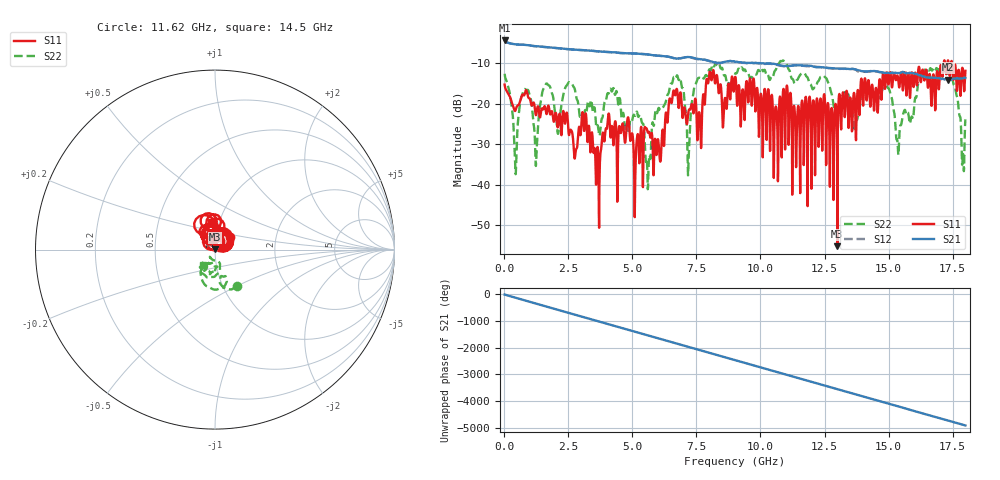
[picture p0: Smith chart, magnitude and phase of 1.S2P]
!Agilent Technologies,E5071C,MY46316741,A.11.02
!Date: Thu Sep 29 15:38:55 2022
!Data & Calibration Information:
!Freq	S11:SOLT2(ON)	S21:SOLT2(ON)	S12:SOLT2(ON)	S22:SOLT2(ON)
!PortZ  Port1:50+j0  Port2:50+j0
!Above PortZ is port z conversion or system Z0 setting when saving the data.
!When reading, reference impedance value at option line is always used.
# Hz S dB R 50
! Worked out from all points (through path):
!   1800 points, 10 MHz to 18 GHz, reference 50 ohm
!   highest |S21| = -4.31 dB at 10 MHz (marker M1); lowest = -14.0 dB at 17.31 GHz (marker M2)
!   group delay of S21, straight-line fit = 758 ps
!   lowest |S11| = -55.3 dB at 13 GHz (marker M3), VSWR 1.00, Z = 50 + j0.169 ohm
!   |S11| at or under -10 dB: start of sweep to 17.15 GHz; 17.21 GHz to 17.3 GHz (89.84 MHz wide, 0.521 % of centre); 17.48 GHz to end of sweep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
!   |S22| runs from -41.2 to -9.3 dB; largest |S21 - S12| = 0.025
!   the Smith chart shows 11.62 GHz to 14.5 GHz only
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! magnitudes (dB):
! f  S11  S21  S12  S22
! 10 MHz  -15.2  -4.3  -4.3  -12.6
! 440 MHz  -21.5  -5.3  -5.3  -37.4
! 830 MHz  -16.8  -5.4  -5.4  -16.5
! 1.23 GHz  -22.8  -5.7  -5.7  -35.4
! 1.65 GHz  -22.6  -5.9  -6.0  -15.0
! 3.01 GHz  -24.5  -6.7  -6.7  -23.0
! 3.64 GHz  -30.7  -7.0  -7.0  -25.3
! 4.31 GHz  -24.9  -7.3  -7.3  -17.6
! 5.61 GHz  -27.2  -7.8  -7.8  -40.6
! 6.01 GHz  -29.1  -8.1  -8.1  -21.2
! 6.66 GHz  -17.8  -8.7  -8.7  -13.6
! 7.18 GHz  -22.3  -8.4  -8.4  -36.5
! 7.54 GHz  -29.0  -8.9  -8.9  -13.9
! 8.08 GHz  -14.1  -9.5  -9.5  -11.4
! 9.01 GHz  -13.3  -9.6  -9.6  -12.6
! 12.01 GHz  -27.0  -10.6  -10.7  -16.1
! 13 GHz  -55.3  -11.2  -11.3  -22.5
! 15.01 GHz  -14.6  -12.3  -12.4  -16.2
! 15.37 GHz  -13.5  -12.4  -12.3  -31.7
! 16.34 GHz  -11.7  -13.2  -13.3  -13.1
! 17.31 GHz  -9.4  -14.0  -14.0  -12.6
! 18 GHz  -11.8  -13.6  -13.7  -23.9
